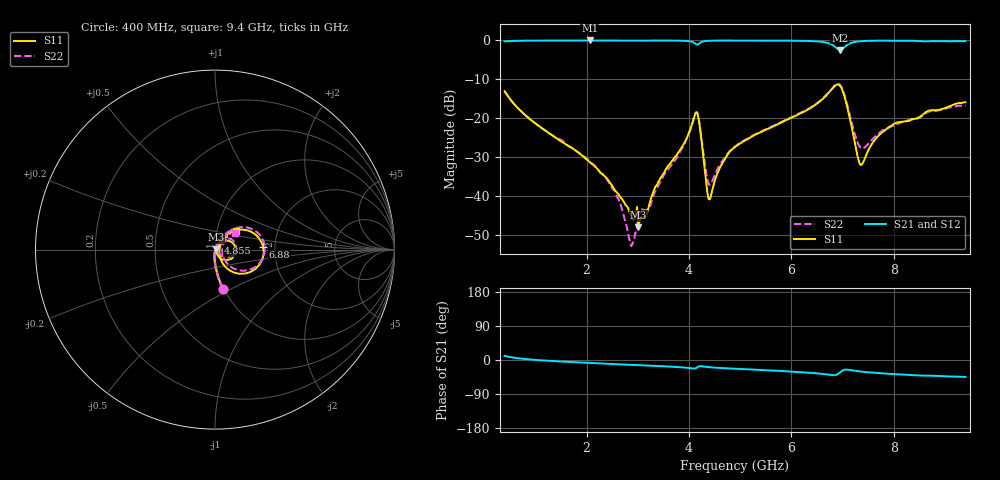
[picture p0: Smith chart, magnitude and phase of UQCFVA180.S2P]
!  Part Number  UQCFVA180  Mounting Orientation: Horizontal
!  Description: Ultra Low ESR Microwave capacitors
!  Application: Coupling, Bypass, Tuning, DC Block
!  Filters, Matching
# GHZ S DB R 50
! Freq  |S11|  S11 Ph  |S21|  S21 Ph  |S12|  S12 Ph  |S22|  S22 Ph
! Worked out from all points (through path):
!   401 points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, 400 MHz to 9.4 GHz, reference 50 ohm
!   highest |S21| = 0.00 dB at 2.065 GHz (marker M1); lowest = -2.5 dB at 6.948 GHz (marker M2)
!   group delay of S21, straight-line fit = 14.7 ps
!   lowest |S11| = -48.2 dB at 3.01 GHz (marker M3), VSWR 1.01, Z = 50.4 + j0.157 ohm
!   |S11| at or under -10 dB: start of sweep to end of sweep
!   |S22| runs from -53.0 to -11.1 dB; largest |S21 - S12| = 0.0026
!   S11 on the Smith chart (normalised r, x): 400 MHz: 0.99, -0.45; 4.855 GHz: 1.04, +0.07; 6.88 GHz: 1.73, +0.06; 9.4 GHz: 1.24, +0.27
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0.4  -13.10 -78.8  -0.22 11.0  -0.23 10.9  -13.09 -79.0
1.908  -29.60 -95.9  -0.01 -6.8  -0.01 -6.8  -29.51 -97.6
2.065  -31.36 -95.4  0.00 -7.9  -0.01 -7.9  -31.12 -99.7
2.583  -39.03 -78.4  -0.02 -11.1  -0.03 -11.1  -39.78 -108.8
2.875  -45.38 -37.9  -0.03 -12.8  -0.03 -12.8  -52.99 -158.2
3.01  -48.18 23.6  -0.04 -13.6  -0.04 -13.6  -44.43 2.1
3.168  -45.09 42.2  -0.05 -14.3  -0.05 -14.3  -43.64 20.5
3.415  -36.13 60.5  -0.02 -15.9  -0.02 -15.9  -37.08 59.8
3.888  -26.95 54.6  -0.07 -19.5  -0.07 -19.6  -27.25 65.0
4.135  -18.62 4.8  -0.94 -21.7  -0.93 -21.7  -18.52 19.0
4.203  -21.34 -44.1  -0.76 -16.4  -0.76 -16.4  -20.96 -28.2
4.338  -36.57 -52.6  -0.14 -18.2  -0.14 -18.2  -34.13 -31.3
4.405  -40.98 4.4  -0.08 -19.1  -0.08 -19.1  -37.22 7.1
4.608  -32.74 57.8  -0.03 -21.0  -0.03 -21.0  -31.89 56.1
4.855  -27.92 60.4  -0.02 -22.7  -0.02 -22.7  -27.70 62.2
4.9  -27.45 60.1  -0.02 -23.0  -0.02 -23.0  -27.26 62.0
6.408  -17.14 46.4  -0.17 -34.0  -0.18 -34.0  -17.03 50.4
6.88  -11.41 3.4  -1.94 -39.0  -1.93 -39.0  -11.23 9.4
6.948  -11.61 -17.8  -2.47 -33.2  -2.46 -33.1  -11.37 -10.7
7.353  -32.04 -10.8  -0.20 -30.4  -0.20 -30.4  -27.59 -11.7
7.915  -22.30 51.6  -0.06 -36.5  -0.06 -36.5  -22.30 40.4
9.4  -15.91 41.6  -0.17 -44.8  -0.17 -44.9  -16.76 39.0
